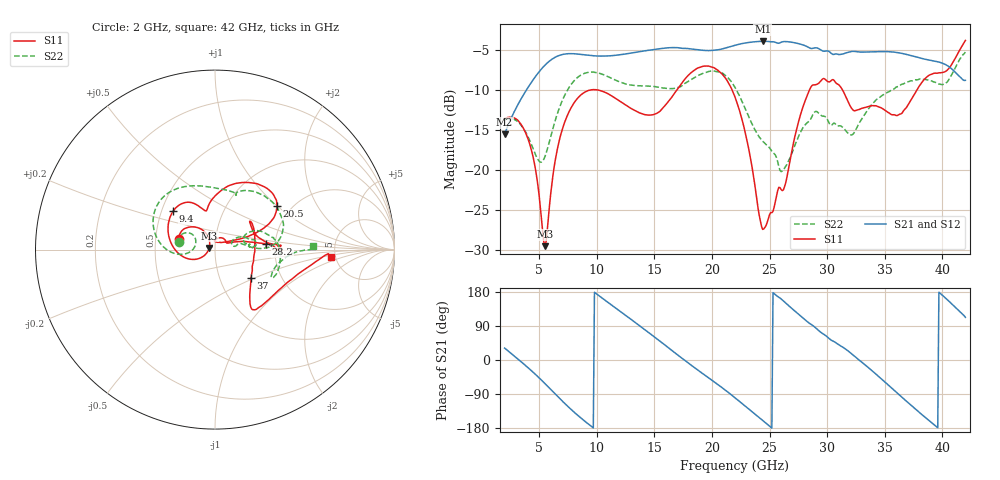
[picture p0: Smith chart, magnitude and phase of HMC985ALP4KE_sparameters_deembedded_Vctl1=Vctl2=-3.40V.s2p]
!s2p File: Measurements: S11, S21, S12, S22
# GHz S dB R 50.0
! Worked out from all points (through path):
!   401 points, 2 GHz to 42 GHz, reference 50 ohm
!   highest |S21| = -3.88 dB at 24.4 GHz (marker M1); lowest = -15.5 dB at 2 GHz (marker M2)
!   lowest |S11| = -29.5 dB at 5.5 GHz (marker M3), VSWR 1.07, Z = 46.9 + j0.808 ohm
!   |S11| at or under -10 dB: start of sweep to 9.338 GHz; 10.21 GHz to 16.93 GHz (6.724 GHz wide, 49.5 % of centre); 21.76 GHz to 28.46 GHz (6.698 GHz wide, 26.7 % of centre)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
!   |S22| runs from -20.2 to -5.2 dB; largest |S21 - S12| = 0.00066
!   S11 on the Smith chart (normalised r, x): 2 GHz: 0.66, +0.08; 9.4 GHz: 0.57, +0.28; 20.5 GHz: 1.69, +1.00; 28.2 GHz: 1.78, +0.13; 37 GHz: 1.41, -0.47; 42 GHz: 4.58, -0.66
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2  -13.53 163.6  -15.51 31.5  -15.51 31.5  -13.68 168.4
4.1  -16.37 127.4  -9.49 -22.1  -9.50 -22.0  -16.02 146.2
5.5  -29.50 165.1  -6.86 -62.1  -6.87 -62.1  -18.32 178.7
6.8  -15.96 -161.4  -5.62 -102.1  -5.61 -102.1  -12.03 -177.4
8.7  -10.49 150.1  -5.53 -155.0  -5.53 -155.0  -8.04 148.6
9.4  -9.98 137.2  -5.65 -172.1  -5.65 -172.1  -7.74 137.1
12.8  -12.13 108.8  -5.39 111.2  -5.39 111.2  -9.32 88.4
15.4  -12.72 100.7  -4.82 51.6  -4.81 51.6  -9.63 69.1
17.8  -8.34 73.5  -4.77 -4.4  -4.76 -4.5  -9.01 66.8
20.5  -7.49 35.0  -4.94 -64.5  -4.94 -64.5  -7.69 26.1
22  -10.84 23.4  -4.38 -99.7  -4.38 -99.7  -9.64 4.9
24.4  -27.41 72.0  -3.88 -159.5  -3.88 -159.5  -16.38 12.5
26.1  -22.56 30.8  -3.94 158.7  -3.95 158.7  -20.12 20.4
28.2  -10.91 6.5  -4.50 103.0  -4.50 103.0  -14.15 17.5
28.7  -9.38 0.9  -4.77 92.2  -4.77 92.1  -13.21 14.8
30.6  -8.76 2.7  -5.51 48.7  -5.51 48.7  -14.10 8.8
32.4  -12.57 26.3  -5.14 9.2  -5.14 9.2  -15.17 23.6
33.9  -11.93 38.0  -5.20 -28.4  -5.20 -28.4  -11.73 24.1
35.4  -12.86 11.5  -5.17 -68.6  -5.17 -68.6  -10.16 14.9
37  -11.88 -37.7  -5.56 -111.9  -5.56 -111.9  -8.95 2.9
39.6  -7.85 -51.9  -6.43 -178.7  -6.44 -178.7  -9.19 -25.6
42  -3.77 -3.7  -8.76 112.4  -8.76 112.4  -5.23 2.1
